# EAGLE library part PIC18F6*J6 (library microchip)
PIC18F97J60 Family 64/80/100-Pin High-Performance, 1-Mbit Flash Microcontrollers with Ethernet Source: http://ww1.microchip.com/downloads/en/DeviceDoc/39762d.pdf
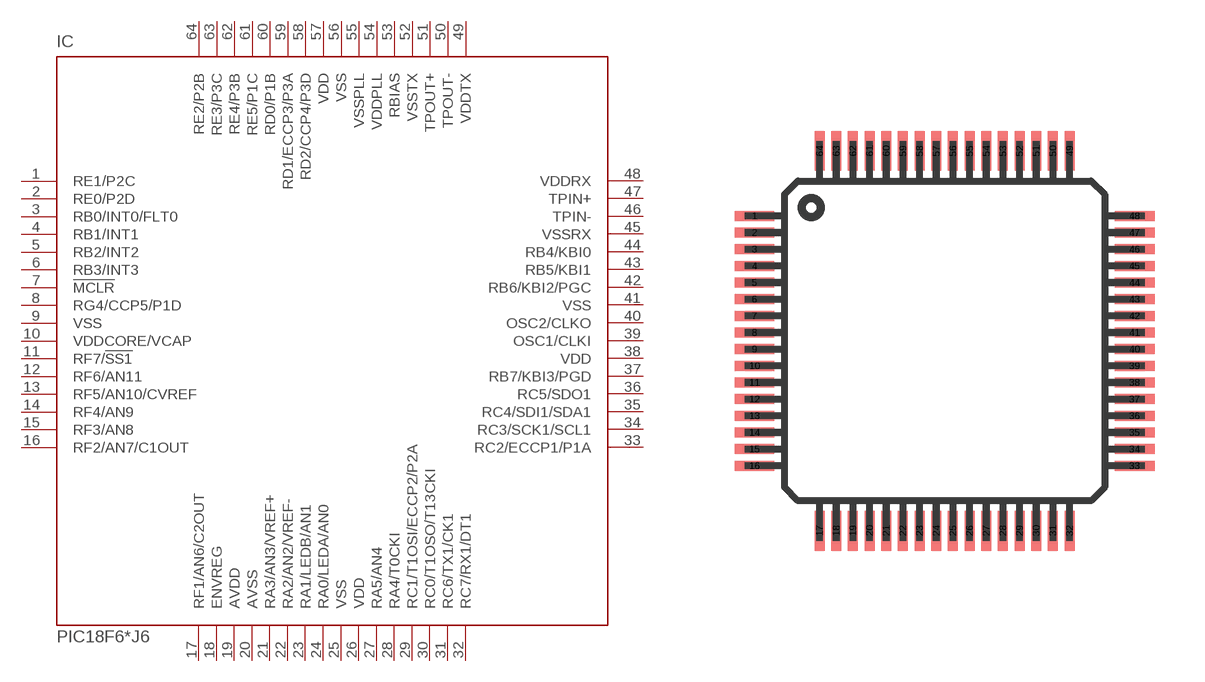
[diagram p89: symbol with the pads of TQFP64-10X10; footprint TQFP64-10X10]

Designator prefix IC

## PIC18F66J60 (MPN: PIC18F66J60-I/PT; OC_FARNELL: 1332282; OC_NEWARK: 56K7296), PIC18F67J60 (MPN: PIC18F67J60-I/PT; OC_FARNELL: 1332285; OC_NEWARK: 56K7302)  [TQFP64-10X10]
1  RE1/P2C
2  RE0/P2D
3  RB0/INT0/FLT0
4  RB1/INT1
5  RB2/INT2
6  RB3/INT3
7  !MCLR
8  RG4/CCP5/P1D
9  VSS
10  VDDCORE/VCAP
11  RF7/!SS1
12  RF6/AN11
13  RF5/AN10/CVREF
14  RF4/AN9
15  RF3/AN8
16  RF2/AN7/C1OUT
17  RF1/AN6/C2OUT
18  ENVREG
19  AVDD
20  AVSS
21  RA3/AN3/VREF+
22  RA2/AN2/VREF-
23  RA1/LEDB/AN1
24  RA0/LEDA/AN0
25  VSS
26  VDD
27  RA5/AN4
28  RA4/T0CKI
29  RC1/T1OSI/ECCP2/P2A
30  RC0/T1OSO/T13CKI
31  RC6/TX1/CK1
32  RC7/RX1/DT1
33  RC2/ECCP1/P1A
34  RC3/SCK1/SCL1
35  RC4/SDI1/SDA1
36  RC5/SDO1
37  RB7/KBI3/PGD
38  VDD
39  OSC1/CLKI
40  OSC2/CLKO
41  VSS
42  RB6/KBI2/PGC
43  RB5/KBI1
44  RB4/KBI0
45  VSSRX
46  TPIN-
47  TPIN+
48  VDDRX
49  VDDTX
50  TPOUT-
51  TPOUT+
52  VSSTX
53  RBIAS
54  VDDPLL
55  VSSPLL
56  VSS
57  VDD
58  RD2/CCP4/P3D
59  RD1/ECCP3/P3A
60  RD0/P1B
61  RE5/P1C
62  RE4/P3B
63  RE3/P3C
64  RE2/P2B

## PIC18F66J65 (MPN: PIC18F66J65-I/PT; OC_FARNELL: 1579612; OC_NEWARK: 56K7298)  [TQFP64-10X10]
Pads as for TQFP64-10X10

## Footprint TQFP64-10X10 (pad centres in mm)
Thin Quad Flat Pack package type TQ
smd 1.2 x 0.3: 1 -5.7,3.75; 2 -5.7,3.25; 3 -5.7,2.75; 4 -5.7,2.25; 5 -5.7,1.75; 6 -5.7,1.25; 7 -5.7,0.75; 8 -5.7,0.25; 9 -5.7,-0.25; 10 -5.7,-0.75; 11 -5.7,-1.25; 12 -5.7,-1.75; 13 -5.7,-2.25; 14 -5.7,-2.75; 15 -5.7,-3.25; 16 -5.7,-3.75; 33 5.7,-3.75; 34 5.7,-3.25; 35 5.7,-2.75; 36 5.7,-2.25; 37 5.7,-1.75; 38 5.7,-1.25; 39 5.7,-0.75; 40 5.7,-0.25; 41 5.7,0.25; 42 5.7,0.75; 43 5.7,1.25; 44 5.7,1.75; 45 5.7,2.25; 46 5.7,2.75; 47 5.7,3.25; 48 5.7,3.75
smd 0.3 x 1.2: 17 -3.75,-5.7; 18 -3.25,-5.7; 19 -2.75,-5.7; 20 -2.25,-5.7; 21 -1.75,-5.7; 22 -1.25,-5.7; 23 -0.75,-5.7; 24 -0.25,-5.7; 25 0.25,-5.7; 26 0.75,-5.7; 27 1.25,-5.7; 28 1.75,-5.7; 29 2.25,-5.7; 30 2.75,-5.7; 31 3.25,-5.7; 32 3.75,-5.7; 49 3.75,5.7; 50 3.25,5.7; 51 2.75,5.7; 52 2.25,5.7; 53 1.75,5.7; 54 1.25,5.7; 55 0.75,5.7; 56 0.25,5.7; 57 -0.25,5.7; 58 -0.75,5.7; 59 -1.25,5.7; 60 -1.75,5.7; 61 -2.25,5.7; 62 -2.75,5.7; 63 -3.25,5.7; 64 -3.75,5.7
